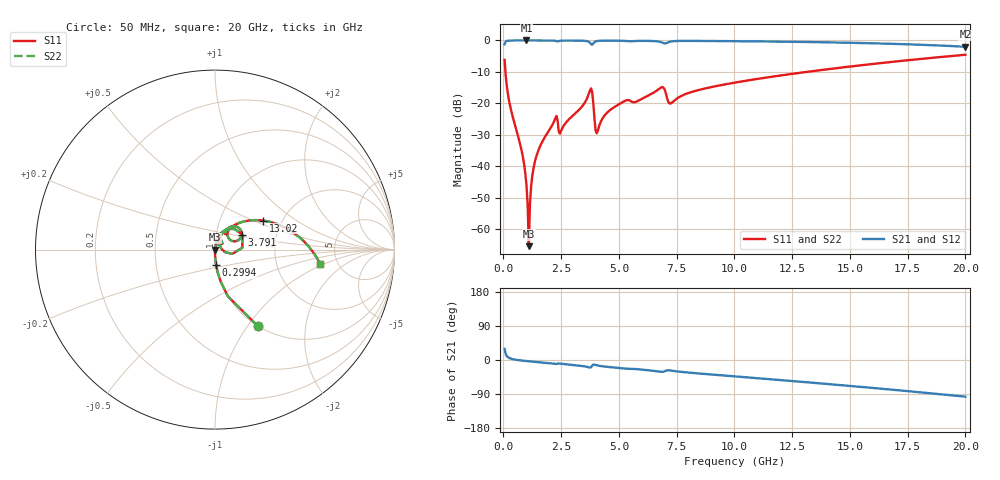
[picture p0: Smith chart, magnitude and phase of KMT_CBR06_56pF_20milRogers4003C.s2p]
! Data measured by Modelithics Inc. support@modelithics.com 813-866-6335
! KEMET CBR0603 56pF, Pad Width= 0.851mm, Pad Length= 0.64mm, Pad Gap= 0.62mm, 20mil Rogers 4003C substrate Data, January 2022
# hz S ma R 50
! 2 Port Network Data from SP1.SP block
! freq  magS11  angS11  magS21  angS21  magS12  angS12  magS22  angS22
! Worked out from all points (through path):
!   401 points, 50 MHz to 20 GHz, reference 50 ohm
!   highest |S21| = 0.00 dB at 997.6 MHz (marker M1); lowest = -2.0 dB at 20 GHz (marker M2)
!   group delay of S21, straight-line fit = 13.6 ps
!   lowest |S11| = -65.5 dB at 1.097 GHz (marker M3), VSWR 1.00, Z = 50.1 + j0.00572 ohm
!   |S11| at or under -10 dB: 86.76 MHz to 13.14 GHz (13.06 GHz wide, 197 % of centre)
!   |S22| runs from -65.5 to -4.6 dB; largest |S21 - S12| = 0
!   S11 on the Smith chart (normalised r, x): 50 MHz: 1.00, -1.13; 299.4 MHz: 1.00, -0.17; 3.791 GHz: 1.34, +0.23; 13.02 GHz: 1.60, +0.57; 20 GHz: 3.66, -0.91
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5e7  0.4913 -60.7  0.8706 29.3  0.8706 29.3  0.4913 -60.7
2.99375e8  0.08716 -85.7  0.9959 4.1  0.9959 4.1  0.08716 -85.7
8.48e8  0.01354 -89.9  0.9994 -1.9  0.9994 -1.9  0.01354 -89.9
9.97625e8  0.004954 -87.1  0.9995 -2.8  0.9995 -2.8  0.004954 -87.1
1.097375e9  0.0005337 6.1  0.9994 -3.4  0.9994 -3.4  0.0005337 6.1
1.197125e9  0.004747 79.3  0.9994 -4.0  0.9994 -4.0  0.004747 79.3
1.34675e9  0.01116 82.1  0.9993 -4.8  0.9993 -4.8  0.01116 82.1
1.695875e9  0.0251 81.5  0.9988 -6.7  0.9988 -6.7  0.0251 81.5
2.2445e9  0.05776 68.7  0.9873 -10.3  0.9873 -10.3  0.05776 68.7
2.493875e9  0.03627 68.8  0.9921 -9.8  0.9921 -9.8  0.03627 68.8
3.391625e9  0.088 71.1  0.991 -15.6  0.991 -15.6  0.088 71.1
3.790625e9  0.1729 28.6  0.8754 -19.2  0.8754 -19.2  0.1729 28.6
3.990125e9  0.03697 4.7  0.9646 -13.1  0.9646 -13.1  0.03697 4.7
4.089875e9  0.03727 47.9  0.9821 -14.6  0.9821 -14.6  0.03727 47.9
4.788125e9  0.08652 67.2  0.9916 -19.9  0.9916 -19.9  0.08652 67.2
6.73325e9  0.1691 50.4  0.959 -30.5  0.959 -30.5  0.1691 50.4
7.232e9  0.0989 40.2  0.9583 -27.7  0.9583 -27.7  0.0989 40.2
1.0025e10  0.2136 45.9  0.9734 -43.3  0.9734 -43.3  0.2136 45.9
1.30175e10  0.3119 31.3  0.9463 -58.1  0.9463 -58.1  0.3119 31.3
1.336662e10  0.3241 29.5  0.9421 -59.9  0.9421 -59.9  0.3241 29.5
1.670825e10  0.4515 11.6  0.8863 -77.7  0.8863 -77.7  0.4515 11.6
2e10  0.592 -7.9  0.794 -96.8  0.794 -96.8  0.592 -7.9
